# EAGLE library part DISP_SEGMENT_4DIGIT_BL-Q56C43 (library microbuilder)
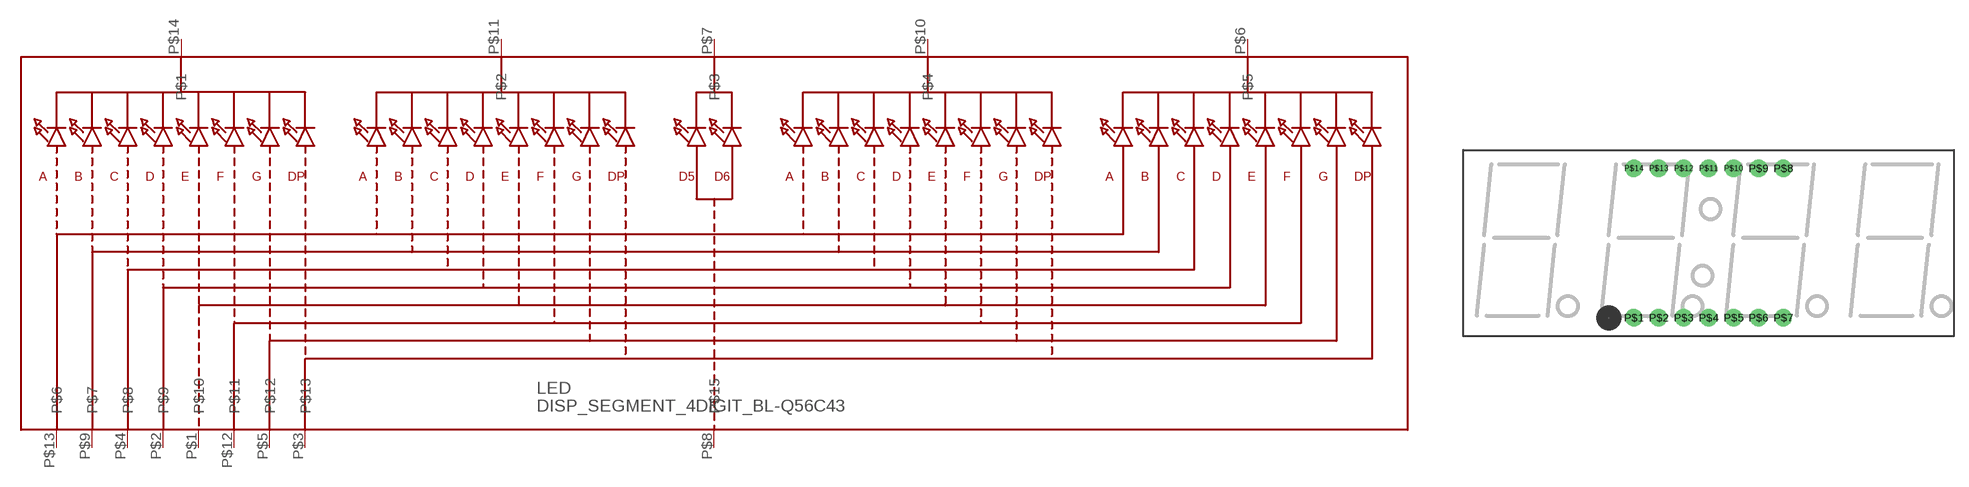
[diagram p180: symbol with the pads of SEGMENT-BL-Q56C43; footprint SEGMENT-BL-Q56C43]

Designator prefix LED

## DISP_SEGMENT_4DIGIT_BL-Q56C43  [SEGMENT-BL-Q56C43]
P$1  P$10
P$2  P$9
P$3  P$13
P$4  P$8
P$5  P$12
P$6  P$5
P$7  P$3
P$8  P$15
P$9  P$7
P$10  P$4
P$11  P$2
P$12  P$11
P$13  P$6
P$14  P$1

## Footprint SEGMENT-BL-Q56C43 (pad centres in mm)
drill 0.8 pad 1.778: P$1 -7.62,-7.62; P$2 -5.08,-7.62; P$3 -2.54,-7.62; P$4 0,-7.62; P$5 2.54,-7.62; P$6 5.08,-7.62; P$7 7.62,-7.62; P$8 7.62,7.62; P$9 5.08,7.62; P$10 2.54,7.62; P$11 0,7.62; P$12 -2.54,7.62; P$13 -5.08,7.62; P$14 -7.62,7.62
